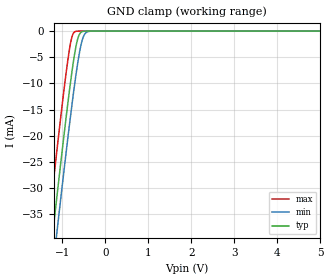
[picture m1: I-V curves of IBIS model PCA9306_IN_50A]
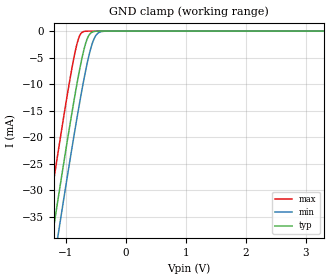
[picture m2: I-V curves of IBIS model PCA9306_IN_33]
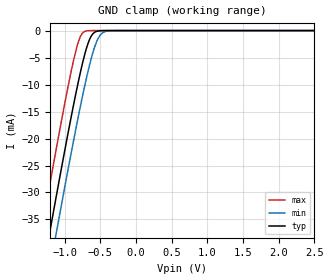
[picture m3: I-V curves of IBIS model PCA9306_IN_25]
| TEXAS INSTRUMENTS INCORPORATED
| Standard Linear and Logic Group
| IBIS Model of PCA9306
| DUAL BIDIRECTIONAL I2C BUS AND SMBUS VOLTAGE-LEVEL TRANSLATOR
| This file contains package information for the following:
|  TSSOP 8-pin (DCT) package as [Component] PCA9306_DCT
|  TSSOP 8-pin (DCU) package as [Component] PCA9306_DCU
| This device can be powered at the following Vccs:
|  5 volt Vcc
|  3.3 volt Vcc
|  2.5 volt Vcc
|  1.8 volt Vcc
|  1.2 volt Vcc
| This file provides unique models under the [Model Selector] for each Vcc.
| For operation at a specific Vcc, select the appropriate model after each
| [Model Selector] keyword.
[IBIS Ver]   3.2
[Comment char]  |_char
[File Name]   pca9306.ibs
[File Rev]   1.2 | x_die
[Date]   April 29, 2009
[Source]   Data created from TI-SPICE simulations at TI-SLL.
[Notes]   The following is an IBIS list for the PCA9306.
   Please contact sllibis@ti.com with questions and
   comments concerning SLL IBIS models.
   - FILE REV HISTORY
   - 1.1 Release IBIS file on 04/19/05
   - Non-monotonic data due to FET characteristics.
   - POWER clamp data deleted as there is no power-clmp diode.
   - 1.2 Release IBIS file on 04/29/09
   - added 2.5V and 1.8V data ranges
[Disclaimer] Property of Texas Instruments Incorporated.  Unauthorized
   reproduction and/or distribution is strictly prohibited.
   This product is protected under copyright law.
   Created  2009, (C) Copyright  2009, Texas Instruments
   Incorporated, All Rights Reserved
   UNLESS THERE IS A SIGNED, WRITTEN AGREEMENT TO THE
   CONTRARY, TEXAS INSTRUMENTS (TI) IS PROVIDING THE IBIS
   MODELS  AND WITHOUT ANY WARRANTY, EXPRESSED OR
   IMPLIED.  TI assumes no liability for:
   1) the accuracy of the IBIS models provided to your
   company;
   2) the proper functioning of these IBIS Models in your
   design or for any resulting applications; or
   3) infringement of patents, copyrights or intellectual
   property rights resulting from your use of these IBIS
   models.
   TI provides IBIS Models as a service to our customers.
   You and your company shall not distribute, sell or give
   these models to anyone else without prior written
   permission from TI.
   TI reserves the right to make changes to our products or
   to discontinue any semiconductor product or service
   without notice, and advises our customers to obtain the
   latest version of relevant information to verify, before
   placing orders, that the information being relied on is
   current.
   Please be aware that your receipt and use of the IBIS
   information provided shall serve as acceptance of these
   terms and conditions.  If you do not accept these terms,
   you should return or destroy the IBIS models and any
   other accompanying information immediately.
| Component PCA9306_DCT 8-PIN TSSOP
[Component]   PCA9306_DCT
[Manufacturer]   Texas Instruments, Inc.
[Package]
|   typ   min   max
R_pkg   2.900e-02   2.800e-02   3.100e-02
L_pkg   1.796e-09   1.666e-09   1.924e-09
C_pkg   1.090e-13   8.300e-14   1.360e-13
[Pin]   signal_name   model_name   R_pin   L_pin   C_pin
1   GND   GND   3.100e-02   1.894e-09   1.340e-13
2   VREF1   PCA9306_IO   2.800e-02   1.697e-09   8.600e-14
3   SCL1   PCA9306_IO   3.000e-02   1.722e-09   8.600e-14
4   SDA1   PCA9306_IO   3.000e-02   1.861e-09   1.300e-13
5   SDA2   PCA9306_IO   2.800e-02   1.924e-09   1.360e-13
6   SCL2   PCA9306_IO   2.900e-02   1.736e-09   8.600e-14
7   VREF2   PCA9306_IO   2.800e-02   1.666e-09   8.300e-14
8   EN   PCA9306_IN   3.000e-02   1.871e-09   1.320e-13
| Component PCA9306_DCU 8-PIN TSSOP
[Component]   PCA9306_DCU
[Manufacturer]   Texas Instruments, Inc.
[Package]
|   typ   min   max
R_pkg   1.400e-02   1.300e-02   1.500e-02
L_pkg   1.289e-09   1.025e-09   2.014e-09
C_pkg   1.360e-13   6.600e-14   2.940e-13
[Pin]   signal_name   model_name   R_pin   L_pin   C_pin
1   GND   GND   1.400e-02   1.387e-09   1.760e-13
2   VREF1   PCA9306_IO   1.300e-02   1.026e-09   6.600e-14
3   SCL1   PCA9306_IO   1.300e-02   1.032e-09   6.700e-14
4   SDA1   PCA9306_IO   1.500e-02   2.014e-09   2.940e-13
5   SDA2   PCA9306_IO   1.400e-02   1.412e-09   1.780e-13
6   SCL2   PCA9306_IO   1.300e-02   1.030e-09   6.600e-14
7   VREF2   PCA9306_IO   1.300e-02   1.025e-09   6.600e-14
8   EN   PCA9306_IN   1.400e-02   1.386e-09   1.760e-13
[Series Switch Groups]
| Function Group States
On  1 /   | VREF1->VREF2 EN HIGH
   | SCL1->SCL2 EN HIGH
   | SDA1->SDA2 EN HIGH
Off 1 /   | EN LOW
[Series Pin Mapping]   pin_2   model_name   function_table_group
2   7   PCA9306_IO_S   1
3   6   PCA9306_IO_S   1
4   5   PCA9306_IO_S   1
| Model PCA9306_IN
[Model Selector]   PCA9306_IN
PCA9306_IN_50A   5 volt Vcc
PCA9306_IN_33   3.3 volt Vcc
PCA9306_IN_25   2.5 volt Vcc
PCA9306_IN_18   1.8 volt Vcc
PCA9306_IN_12A   1.2 volt Vcc
| Model PCA9306_IO
[Model Selector]   PCA9306_IO
PCA9306_IO_50A   5 volt Vcc
PCA9306_IO_33   3.3 volt Vcc
PCA9306_IO_25   2.5 volt Vcc
PCA9306_IO_18   1.8 volt Vcc
PCA9306_IO_12A   1.2 volt Vcc
| Model PCA9306_IO_S
[Model Selector]   PCA9306_IO_S
PCA9306_IO_50A_S   5 volt Vcc
PCA9306_IO_33_S   3.3 volt Vcc
PCA9306_IO_25_S   2.5 volt Vcc
PCA9306_IO_18_S   1.8 volt Vcc
PCA9306_IO_12A_S   1.2 volt Vcc
[Model]   PCA9306_IO_50A_S
Model_type  Series_switch
| variable   typ   min   max
C_comp   0   0   0
[Temperature Range]   40   100   -40
| Ambient temperature   25   85   -40
[Voltage range]   5   5   5
[On]
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[Off]
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[Model]   PCA9306_IO_33_S
Model_type  Series_switch
| variable   typ   min   max
C_comp   0   0   0
[Temperature Range]   40   100   -40
| Ambient temperature   25   85   -40
[Voltage range]   3.3   3   3.6
[On]
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[Off]
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[Model]   PCA9306_IO_25_S
Model_type  Series_switch
| variable   typ   min   max
C_comp   0   0   0
[Temperature Range]   40   100   -40
| Ambient temperature   25   85   -40
[Voltage range]   2.5   2.3   2.7
[On]
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[Off]
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[Model]   PCA9306_IO_18_S
Model_type  Series_switch
| variable   typ   min   max
C_comp   0   0   0
[Temperature Range]   40   100   -40
| Ambient temperature   25   85   -40
[Voltage range]   1.8   1.65   1.95
[On]
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[Off]
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[Model]   PCA9306_IO_12A_S
Model_type  Series_switch
| variable   typ   min   max
C_comp   0   0   0
[Temperature Range]   40   100   -40
| Ambient temperature   25   85   -40
[Voltage range]   1.2   1.2   1.2
[On]
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[Off]
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| Models and submodels in the file (15): PCA9306_IN_50A (Input), PCA9306_IN_33 (Input), PCA9306_IN_25 (Input), PCA9306_IN_18 (Input), PCA9306_IN_12A (Input), PCA9306_IO_50A_S (Series_switch), PCA9306_IO_50A (Terminator), PCA9306_IO_33_S (Series_switch), PCA9306_IO_33 (Terminator), PCA9306_IO_25_S (Series_switch), PCA9306_IO_25 (Terminator), PCA9306_IO_18_S (Series_switch), PCA9306_IO_18 (Terminator), PCA9306_IO_12A_S (Series_switch), PCA9306_IO_12A (Terminator)
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[Model]   PCA9306_IN_50A
Model_type  Input
Vinl=0.6
Vinh=5
| variable   typ   min   max
C_comp   6.26pF   4.66pF   9.23pF
[Temperature Range]   40   100   -40
| Ambient temperature   25   85   -40
[Voltage range]   5   5   5
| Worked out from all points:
|   GND clamp passes 1 mA (typ) near -0.62 V on its own axis
[GND Clamp]
| PCA9306_IN_50A
|   Voltage   I(typ)   I(min)   I(max)
-5V       -328.9mA   -335.1mA   -321mA
-1.365V   -49.02mA   -55.82mA   -40.25mA
-1.325V   -46.04mA   -52.85mA   -37.26mA
-1.215V   -37.92mA   -44.74mA   -29.12mA
-1.12V    -30.99mA   -37.81mA   -22.19mA
-850mV    -12.22mA   -18.79mA   -4.2mA
-780mV    -7.858mA   -14.16mA   -1.166mA
-710mV    -4.062mA   -9.799mA   -118uA
-635mV    -1.238mA   -5.618mA   -5.709uA
-555mV    -167.5uA   -2.206mA   -200.7nA
-405mV    -1.746uA   -97.01uA   -397.3pA
5V        97.63pA    2.873nA    90.01pA
[Model]   PCA9306_IN_33
Model_type  Input
Vinl=0.6
Vinh=3.6
| variable   typ   min   max
C_comp   6.06pF   4.74pF   7.90pF
[Temperature Range]   40   100   -40
| Ambient temperature   25   85   -40
[Voltage range]   3.3   3   3.6
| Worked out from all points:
|   GND clamp passes 1 mA (typ) near -0.62 V on its own axis
[GND Clamp]
| PCA9306_IN_33
|   Voltage   I(typ)   I(min)   I(max)
-3.3V     -197mA     -203.5mA   -188.9mA
-1.36V    -48.65mA   -55.45mA   -39.88mA
-1.315V   -45.3mA    -52.12mA   -36.52mA
-1.23V    -39.02mA   -45.85mA   -30.22mA
-1.19V    -36.09mA   -42.91mA   -27.28mA
-1.115V   -30.63mA   -37.45mA   -21.83mA
-850mV    -12.22mA   -18.79mA   -4.2mA
-715mV    -4.305mA   -10.1mA    -142.6uA
-635mV    -1.238mA   -5.618mA   -5.709uA
-555mV    -167.5uA   -2.206mA   -200.7nA
-405mV    -1.746uA   -97.01uA   -397.3pA
3.3V      64.05pA    2.84nA     56.56pA
[Model]   PCA9306_IN_25
Model_type  Input
Vinl=0.6
Vinh=2.7
| variable   typ   min   max
C_comp   5.97pF   4.76pF   7.97pF
[Temperature Range]   40   100   -40
| Ambient temperature   25   85   -40
[Voltage range]   2.5   2.3   2.7
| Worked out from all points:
|   GND clamp passes 1 mA (typ) near -0.62 V on its own axis
[GND Clamp]
| PCA9306_IN_25
|   Voltage   I(typ)   I(min)   I(max)
-2.5V     -135.3mA   -141.9mA   -127mA
-1.335V   -46.79mA   -53.6mA    -38.01mA
-1.22V    -38.29mA   -45.11mA   -29.48mA
-1.185V   -35.72mA   -42.55mA   -26.92mA
-1.12V    -30.99mA   -37.81mA   -22.19mA
-855mV    -12.54mA   -19.12mA   -4.472mA
-785mV    -8.155mA   -14.49mA   -1.319mA
-720mV    -4.553mA   -10.4mA    -171.8uA
-640mV    -1.37mA    -5.873mA   -7.034uA
-560mV    -192.8uA   -2.373mA   -247.3nA
-415mV    -2.384uA   -124.1uA   -599.6pA
2.5V      48.96pA    2.825nA    41.29pA
